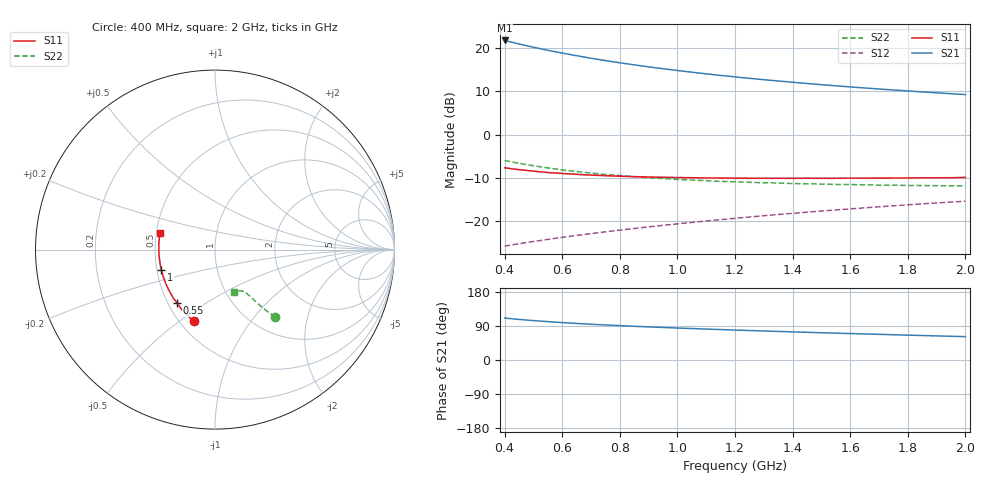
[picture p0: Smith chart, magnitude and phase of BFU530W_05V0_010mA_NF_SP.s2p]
! Filename:  P:\Prog\Test\Noise\ATS_data\Testdata_Net\06 Compressed Noise after Statistics\BFU530W_APM2013_09_A05_05p0V_010mA_NF_CM01_D.sf
! Date/Time: Tue 26/Mar/2013 18:06:05
! BFU530W_APM2013_09_A05_05p0V_1to25mA_NF_CM01_Bias6_R.sf
! Noise Parameter Data File
! BFU530W_APM2013_09_A05_05p0V_1to25mA_NF_CM01
! Date/time: Thu Mar 21 20:31:54 2013
! VAR V_out= 5.000000
! VAR I_out= 9.995000
! VAR V_in= 0.828400
! VAR I_in= 0.105305
! Device data file deembeded for feedlines and parallel
! Original file: \06 Compressed Noise after Statistics\BFU530W_APM2013_09_A05_05p0V_010mA_NF_CM01_R.sf
! Feed-files: PR019V01_070313_Feed1.s2p, PR019V01_070313_Feed2.s2p
! Parallel-file: PR019V01_070313_Par.s2p
# MHz S MA R 50
!  Freq-MHz  S11-mag  S11-arg  S21-mag  S21-arg  S12-mag  S12-arg  S22-mag  S22-arg
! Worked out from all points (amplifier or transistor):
!   37 points, 400 MHz to 2 GHz, reference 50 ohm
!   highest |S21| = 21.8 dB at 400 MHz (marker M1)
!   |S21| within 3 dB of that: start of sweep to 607.2 MHz
!   unconditionally stable (mu >= 1): 1.342 GHz to end of sweep
!   at 500 MHz: K = 0.73, MSG = 22.5 dB, |S12| = -24.7 dB
!   at 1.1 GHz: K = 0.97, MSG = 17.0 dB, |S12| = -20.0 dB
!   at 2 GHz: K = 1.02, MAG = 11.4 dB, |S12| = -15.4 dB
!   lowest NFmin = 0.75 dB at 480 MHz
!   S11 on the Smith chart (normalised r, x): 400 MHz: 0.59, -0.56; 550 MHz: 0.56, -0.38; 1 GHz: 0.53, -0.13; 2 GHz: 0.52, +0.11
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400  0.4136 -106.7  12.27 110.7  0.05143 59.0  0.5023 -48.0
420  0.4057 -109.7  11.82 109.2  0.05287 59.0  0.4874 -48.6
433  0.4 -111.5  11.53 108.3  0.05375 59.0  0.4781 -48.9
460  0.3913 -115.0  10.98 106.5  0.05561 59.1  0.4612 -49.5
500  0.3788 -120.1  10.24 104.0  0.05819 59.3  0.4371 -50.2
550  0.3648 -125.4  9.459 101.2  0.06164 59.8  0.4129 -50.8
600  0.3564 -130.6  8.779 98.7  0.06505 60.2  0.3917 -51.3
650  0.3478 -135.2  8.177 96.5  0.06846 60.6  0.3751 -51.8
700  0.3411 -139.5  7.651 94.4  0.07185 61.1  0.3602 -52.2
750  0.3357 -143.3  7.187 92.5  0.0753 61.5  0.347 -52.4
800  0.3307 -147.0  6.777 90.7  0.07885 62.0  0.337 -52.9
850  0.3274 -150.5  6.41 89.0  0.08235 62.3  0.3265 -53.1
950  0.3216 -156.4  5.787 85.8  0.08955 63.1  0.3113 -53.8
1000  0.3196 -159.3  5.518 84.4  0.09316 63.3  0.3039 -54.0
1100  0.3161 -164.4  5.049 81.6  0.1005 63.8  0.2939 -54.9
1200  0.3141 -169.2  4.657 79.0  0.108 64.1  0.2857 -55.7
1250  0.3135 -171.4  4.48 77.8  0.1117 64.2  0.2813 -56.1
1350  0.313 -175.2  4.174 75.4  0.1195 64.4  0.2758 -57.1
1500  0.313 179.0  3.784 71.9  0.131 64.4  0.2686 -59.0
1600  0.3145 175.5  3.564 69.8  0.1388 64.4  0.2651 -60.1
1750  0.3155 170.8  3.287 66.7  0.1506 64.1  0.2606 -62.0
2000  0.3204 163.5  2.908 61.6  0.1704 63.4  0.256 -66.0
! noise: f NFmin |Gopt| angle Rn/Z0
400  0.7532  0.08836  158.4  0.0791
460  0.7723  0.08948  162.6  0.0787
600  0.7852  0.08898  160.3  0.082
800  0.8177  0.1199  166.5  0.0769
1000  0.8375  0.1337  169.9  0.0771
1200  0.9058  0.1505  172.2  0.0758
1400  0.9086  0.175  175.9  0.0738
1600  0.9116  0.2157  179.2  0.066
1800  0.9423  0.2273  -173.7  0.0707
2000  0.977  0.2469  -171.3  0.0698
